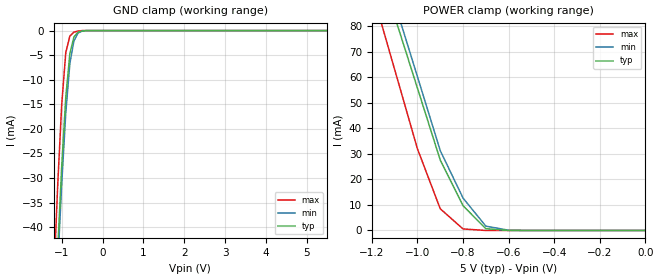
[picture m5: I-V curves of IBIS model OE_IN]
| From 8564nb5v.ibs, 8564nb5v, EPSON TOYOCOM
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[Model]   OE_IN
Model_type   Input
Polarity   Non-Inverting
Vinl =   1.5V
Vinh =   3.5V
C_comp   5pF   5pF   5pF
[Temperature Range]   25.00   85.00   -40.00
[Voltage Range]   5.0V   4.5V   5.50V
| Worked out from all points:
|   GND clamp passes 1 mA (typ) near -0.67 V on its own axis
|   POWER clamp passes 1 mA (typ) near -0.70 V on its own axis
[GND_clamp]
| voltage   I(typ)   I(min)   I(max)
-5.5V     -932.7mA   -905.3mA   -921mA
-1.2V     -64.1mA    -66.8mA    -52mA
-1.1V     -45.1mA    -48.4mA    -31.9mA
-1V       -27.7mA    -31.3mA    -15.1mA
-900mV    -13.6mA    -16.8mA    -4.5mA
-800mV    -4.7mA     -6.7mA     -1.1mA
-700mV    -1.3mA     -2.1mA     -300uA
-600mV    -300uA     -500uA     -100uA
-500mV    -100uA     -100uA     0A
-400mV    0A         0A         0A
5.5V      0A         0A         0A
[POWER_clamp]
| voltage   I(typ)   I(min)   I(max)
-5.5V     1.323A     1.363A     1.433A
-1.2V     112.1mA    118.1mA    94.3mA
-1.1V     83.9mA     89.2mA     63.1mA
-1V       55.8mA     60.3mA     32mA
-900mV    27.6mA     31.3mA     8.5mA
-800mV    9.7mA      12.7mA     600uA
-700mV    700uA      1.7mA      0A
-600mV    0A         100uA      0A
0V        0A         0A         0A
